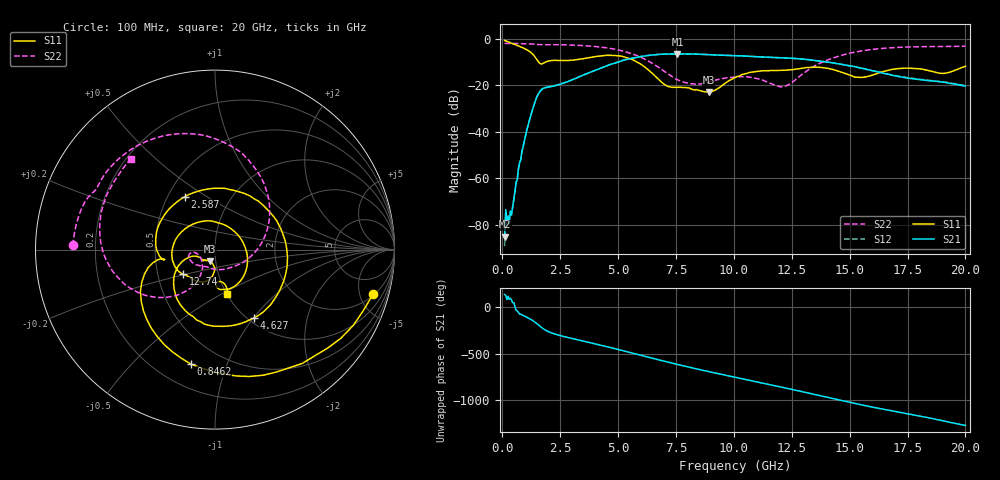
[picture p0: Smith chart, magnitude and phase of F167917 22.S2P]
!  2-Port S-parameters saved by WinCal
! VAR MeasName=S-Parameters (CALIBRATED_DATA) read from VNA (N5242A)
! VAR MeasDate=2016-11-22 9:00:48
! VAR NAME=F167917 22
! VAR FILENAME=F167917 22.S2P
! VAR DATE=2016-11-22 9:00:48
! VAR PHYS_PORTS=1,2
# Hz S DB R 50
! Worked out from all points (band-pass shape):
!   401 points, 100 MHz to 20 GHz, reference 50 ohm
!   highest |S21| = -6.56 dB at 7.562 GHz (marker M1); lowest = -85.1 dB at 100 MHz (marker M2)
!   |S21| within 3 dB of the highest: 5.144 GHz to 13.67 GHz (8.522 GHz wide, 90.6 % of centre)
!   lowest |S11| = -23.0 dB at 8.906 GHz (marker M3), VSWR 1.15, Z = 46.8 - j6.11 ohm
!   |S11| at or under -10 dB: 1.563 GHz to 1.886 GHz (322.2 MHz wide, 18.7 % of centre); 5.815 GHz to end of sweep
!   |S22| runs from -20.7 to -2.0 dB; largest |S21 - S12| = 0.0051
!   S11 on the Smith chart (normalised r, x): 100 MHz: 2.18, -6.64; 846.2 MHz: 0.34, -0.75; 2.587 GHz: 0.61, +0.40; 4.627 GHz: 1.07, -1.01; 12.74 GHz: 0.68, -0.20; 20 GHz: 1.01, -0.53
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1e8  -0.76 -15.5  -85.11 137.1  -89.24 -152.8  -2.03 178.3
3.985e8  -1.95 -52.6  -75.72 77.2  -75.92 74.1  -2.06 173.4
8.4625e8  -3.72 -101.9  -48.60 -80.4  -48.53 -79.8  -2.14 166.2
1.1945e9  -5.62 -139.7  -34.20 -125.1  -34.13 -124.8  -2.23 160.4
1.5925e9  -10.37 -170.3  -23.20 163.3  -23.13 163.2  -2.53 154.2
2.5875e9  -9.38 119.9  -19.30 49.9  -19.27 49.6  -2.62 138.8
3.43325e9  -8.71 38.4  -15.93 0.1  -15.92 -0.0  -2.94 121.7
4.03025e9  -7.68 -13.9  -13.49 -34.6  -13.48 -34.5  -3.39 107.5
4.62725e9  -7.15 -60.1  -11.23 -69.9  -11.21 -69.9  -4.14 90.8
5.672e9  -9.26 -128.4  -8.31 -136.2  -8.26 -136.3  -6.74 53.9
6.7665e9  -17.65 -163.6  -6.75 153.9  -6.75 153.7  -12.44 1.2
7.5625e9  -20.90 -139.5  -6.56 105.2  -6.58 105.1  -17.66 -51.5
8.90575e9  -22.95 -114.1  -6.87 28.7  -6.86 28.6  -18.58 -128.1
1.005e10  -16.78 -95.3  -7.31 -32.5  -7.30 -32.4  -16.55 -156.2
1.129375e10  -13.79 -120.5  -7.93 -98.3  -7.88 -98.2  -18.03 -173.4
1.208975e10  -13.62 -132.4  -8.24 -140.5  -8.18 -140.7  -20.70 -150.1
1.27365e10  -13.00 -142.1  -8.60 -176.0  -8.57 -176.1  -16.98 -121.4
1.338325e10  -12.28 -160.5  -9.21 147.5  -9.20 147.5  -12.32 -121.6
1.5025e10  -15.71 101.9  -11.72 57.4  -11.73 57.5  -6.21 -150.6
1.67165e10  -13.46 -37.9  -15.40 -29.4  -15.38 -28.4  -3.95 177.4
1.905475e10  -14.95 -82.0  -18.71 -141.4  -18.59 -141.5  -3.38 143.8
2e10  -11.85 -74.3  -20.37 169.1  -20.18 169.2  -3.24 132.8
